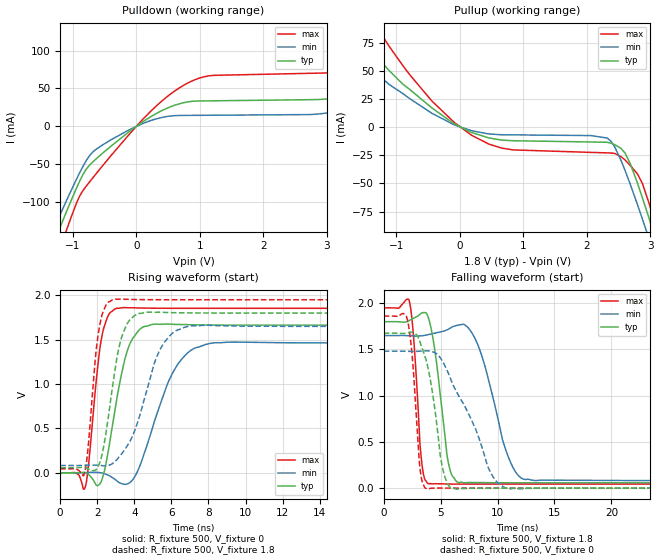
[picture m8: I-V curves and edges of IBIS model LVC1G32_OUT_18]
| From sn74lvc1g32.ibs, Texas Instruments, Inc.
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[Model]   LVC1G32_OUT_18
Model_type  Output
Vref =   0.0
Rref =   1000
Cref =   30p
Vmeas =   0.9
| variable   typ   min   max
C_comp   8.02pF   0.98pF   15.78pF
| C_pullup   5.15pF   0.98pF   7.82pF
| C_pulldown   10.88pF   6.80pF   15.78pF
[Temperature Range]   40   100   -40
| Ambient temperature   25   85   -40
[Voltage range]   1.8   1.65   1.95
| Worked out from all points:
|   slope of the pulldown table from 0 to 0.27 V, typ, clamps not added: 18.2 ohm
|   slope of the pullup table from 0 to 0.27 V, typ, clamps not added: 40.8 ohm
|   rising waveform, R_fixture 500, V_fixture 0: 20-80 % time 892ps typ, 1.53ns min, 545ps max; typ from 0 V to 1.66 V
|   rising waveform, R_fixture 500, V_fixture 1.8: 20-80 % time 779ps typ, 1.41ns min, 494ps max; typ from 0.058 V to 1.8 V
|   falling waveform, R_fixture 500, V_fixture 1.8: 20-80 % time 980ps typ, 1.92ns min, 559ps max; typ from 1.8 V to 0.058 V
|   falling waveform, R_fixture 500, V_fixture 0: 20-80 % time 1.17ns typ, 3.12ns min, 625ps max; typ from 1.68 V to 0 V
[Pulldown]
| LVC1G32_OUT_18
|   Voltage   I(typ)   I(min)   I(max)
-5V       -926.2mA   -845.6mA   -1.059A
-1.285V   -150.6mA   -132.2mA   -181mA
-1.13V    -118.6mA   -103.4mA   -143.9mA
-645mV    -43.82mA   -30.94mA   -63.68mA
120mV     7.037mA    4.343mA    10.87mA
790mV     31.99mA    14.4mA     56.3mA
3.325V    41.15mA    22.83mA    73.35mA
4.18V     65.15mA    16.29mA    106.5mA
4.445V    38.68mA    16.42mA    121.1mA
4.7V      37.61mA    16.54mA    131.5mA
5.1V      37.87mA    16.73mA    75.58mA
10V       42.22mA    18.93mA    82.87mA
[Pullup]
| LVC1G32_OUT_18
|   Voltage   I(typ)   I(min)   I(max)
-5V       376.5mA    301.6mA    519.2mA
-2.1V     117.1mA    90.82mA    164.6mA
-1.62V    82.48mA    63.2mA     116.7mA
-1.12V    50.56mA    38.12mA    72.26mA
-440mV    17.01mA    12.27mA    23.14mA
455mV     -9.587mA   -6.043mA   -15.04mA
2.32V     -13.48mA   -9.703mA   -22.88mA
2.6V      -22.99mA   -38.43mA   -29.17mA
2.795V    -49.58mA   -68.71mA   -41.49mA
2.98V     -81.29mA   -99.53mA   -67.98mA
3.15V     -112.1mA   -128.9mA   -100.8mA
10V       -1.513A    -1.437A    -1.648A
[Ramp]
| LVC1G32_OUT_18
| variable   typ   min   max
dV/dt_r   1.09/9.73E-10   0.96/1.73E-09   1.23/6.09E-10
dV/dt_f   1.10/1.07E-09   1.01/2.24E-09   1.20/6.20E-10
R_load = 500
[Rising Waveform]
| LVC1G32_OUT_18
R_fixture =   500
C_fixture =   0
L_fixture =   0
V_fixture =   0
V_fixture_min = 0
V_fixture_max = 0
|   Time   V(typ)   V(min)   V(max)
0s        -10.92uV   -1.519uV   -22.17uV
1.35ns    2.342mV    1.686mV    -163.7mV
2.225ns   -93.41mV   -1.451mV   1.509V
2.595ns   243.5mV    -27.97mV   1.773V
3.06ns    837.2mV    -90.67mV   1.854V
3.655ns   1.394V     -122.6mV   1.859V
4.365ns   1.628V     113.3mV    1.857V
6.2ns     1.672V     1.174V     1.853V
8.155ns   1.665V     1.461V     1.853V
50ns      1.664V     1.463V     1.853V
[Rising Waveform]
| LVC1G32_OUT_18
R_fixture =   500
C_fixture =   0
L_fixture =   0
V_fixture =   1.8
V_fixture_min = 1.65
V_fixture_max = 1.95
|   Time   V(typ)   V(min)   V(max)
0s        57.97mV    82.43mV    43.9mV
1.31ns    61.47mV    83.75mV    -10.01mV
2.09ns    90.03mV    84.49mV    1.609V
2.45ns    418.5mV    78.45mV    1.88V
2.92ns    1.102V     119.8mV    1.956V
3.35ns    1.548V     222.5mV    1.957V
3.99ns    1.767V     458.2mV    1.952V
5.42ns    1.809V     1.401V     1.95V
6.98ns    1.802V     1.653V     1.95V
50ns      1.8V       1.65V      1.95V
[Falling Waveform]
| LVC1G32_OUT_18
R_fixture =   500
C_fixture =   0
L_fixture =   0
V_fixture =   1.8
V_fixture_min = 1.65
V_fixture_max = 1.95
|   Time   V(typ)   V(min)   V(max)
0s        1.8V       1.65V      1.95V
2.25ns    1.812V     1.648V     2.022V
3.305ns   1.892V     1.647V     316.6mV
3.935ns   1.838V     1.661V     46.69mV
5.62ns    312mV      1.716V     44.78mV
6.55ns    60.43mV    1.764V     43.76mV
8.19ns    60.81mV    1.574V     43.69mV
10.73ns   58.08mV    411.8mV    43.89mV
12.29ns   57.92mV    96.74mV    43.92mV
50ns      57.97mV    82.46mV    43.9mV
[Falling Waveform]
| LVC1G32_OUT_18
R_fixture =   500
C_fixture =   0
L_fixture =   0
V_fixture =   0
V_fixture_min = 0
V_fixture_max = 0
|   Time   V(typ)   V(min)   V(max)
0s        1.675V     1.481V     1.861V
2.085ns   1.679V     1.48V      1.82V
2.52ns    1.686V     1.479V     1.401V
3.17ns    1.587V     1.481V     232.7mV
3.69ns    1.399V     1.485V     -3.086mV
5.11ns    254.3mV    1.383V     629.2uV
5.935ns   2.665mV    1.162V     -59.1uV
9.38ns    106.4uV    170.4mV    -28.51uV
10.88ns   -19.43uV   -4.551mV   -1.855uV
50ns      -6.377uV   13.53uV    -21.57uV
